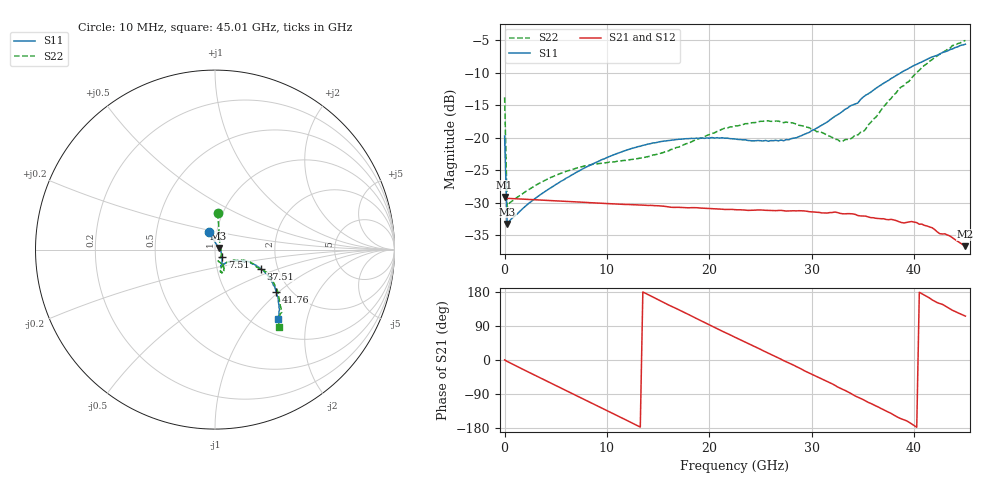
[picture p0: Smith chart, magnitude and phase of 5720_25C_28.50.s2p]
! Device:  ADRF5720
! Description: 0.5dB LSB GaAs MMIC 6-bit Digital Attenuator
! Frequency:  0.000009 -  40 GHz
! Ports:
!	RF1	= Port 1
!	RF2	= Port 2
! Vdd:  3.3 Volt
! Vss:  -3.3 Volt
! Control:  0/3.3 Volt
! State:  28.50 dB attenuation
! Data:  The device was measured using G-S-G Probes on a matrix board.
!  Data was collected using an calibrated 4 port network analyzer.
!  The reference plane for this measurement is at the launchers.
! Note:  Analog Devices supplies this data as a sample of measured data
!  for this product.  Your particular data for this product may vary.
!  Data was taken at 25 degrees C.
!  Analog Devices reserves the right to change this data at anytime.
# GHZ S DB R 45.0
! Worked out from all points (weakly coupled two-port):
!   181 points, 10 MHz to 45.01 GHz, reference 45 ohm
!   highest |S21| = -29.10 dB at 10 MHz (marker M1); lowest = -36.6 dB at 45.01 GHz (marker M2)
!   lowest |S11| = -33.2 dB at 260 MHz (marker M3), VSWR 1.04, Z = 46.8 + j0.873 ohm
!   |S11| at or under -10 dB: start of sweep to 38.74 GHz
!   |S22| runs from -30.6 to -5.1 dB; largest |S21 - S12| = 0.00013
!   S11 on the Smith chart (normalised r, x): 10 MHz: 0.92, +0.18; 7.51 GHz: 1.08, -0.09; 37.51 GHz: 1.63, -0.37; 41.76 GHz: 1.69, -0.97; 45.01 GHz: 1.27, -1.35
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0.01  -19.73 109.2  -29.10 0.2  -29.10 0.2  -13.79 85.6
0.26  -33.24 25.4  -29.30 -3.7  -29.31 -3.7  -30.62 15.6
3.26  -29.01 -19.0  -29.53 -44.2  -29.53 -44.2  -27.10 -35.2
7.51  -24.89 -46.2  -29.89 -100.5  -29.89 -100.4  -24.47 -67.3
7.76  -24.68 -47.3  -29.91 -103.8  -29.91 -103.8  -24.36 -68.5
12.01  -21.85 -61.2  -30.24 -160.2  -30.24 -160.2  -23.46 -74.4
15.26  -20.59 -67.7  -30.48 155.6  -30.48 155.6  -22.38 -68.8
20.26  -19.97 -71.3  -30.88 89.2  -30.88 89.2  -19.35 -63.6
22.76  -20.26 -69.2  -31.06 56.8  -31.06 56.8  -18.19 -66.4
25.51  -20.42 -59.6  -31.14 21.3  -31.13 21.3  -17.40 -71.8
27.26  -20.47 -51.5  -31.20 -1.6  -31.19 -1.5  -17.69 -74.3
30.26  -18.74 -33.6  -31.40 -40.8  -31.41 -40.7  -18.81 -74.5
32.76  -16.25 -24.1  -31.60 -74.2  -31.60 -74.2  -20.56 -60.0
33.76  -15.12 -22.6  -31.66 -87.3  -31.65 -87.3  -20.20 -46.3
34.51  -14.67 -20.6  -31.94 -98.2  -31.92 -98.1  -19.58 -38.8
35.01  -13.79 -20.2  -32.01 -104.3  -32.01 -104.2  -19.13 -33.1
37.51  -11.20 -22.6  -32.58 -137.7  -32.57 -137.6  -14.32 -19.9
37.76  -10.92 -23.1  -32.52 -141.0  -32.51 -141.1  -13.97 -19.6
40.26  -8.74 -29.7  -33.03 -177.5  -33.00 -177.4  -9.98 -23.8
41.76  -7.61 -34.7  -33.81 158.7  -33.81 159.0  -8.02 -31.8
43.76  -6.37 -42.1  -35.37 131.0  -35.37 131.0  -5.84 -43.0
45.01  -5.65 -47.8  -36.64 115.8  -36.69 115.7  -5.08 -50.4
